| Texas Instruments Incorporated
| USB 3.0 xHCI Host Controller
| Marketing part#   Voltage Range   Package-type   Temperature
| TUSB7340   2.97V - 3.465V   100-Ball RKM QFN   -40 to 105 C
| TUSB7320   2.97V - 3.465V   100-Ball RKM QFN   -40 to 105 C
[IBIS Ver]   4.0
[File name]   tusb7340_20.ibs
[File Rev]   1.0
[Date]   12/02/2010
[Source]   Model built from TISPICE simulations at:
   Texas Instruments Incorporated.
   Analog-eLab, HPA
   12500 TI Blvd
   Dallas, TX -75243
   For Support e-mail: elab_scm_ibis@list.ti.com
[Notes]   Rev 1.0: 12/02/2010
   - Model based on tusb1310.ibs v1.1 09/14/2010 IBIS model.
   - Model generated from simulations in TISPICED
   - For USB2.0, models are included for HS, FS and LS modes
   - For USB3.0, models are included for SATA1, SATA2, No-De-Emphasis
   and De-Emphasis modes
   - USB2 and USB3 Models  matched to TISPICE.
   - C_comp although listed in numerical order of value are obtained from varying
   PVT conditions. For PVT conditions for each specific value refer the buffer
   description under respective [Model]. IBIS model user is responsible for using
   appropriate C_comp to simulate for Signal Integrity
   Where for TUSB7340 & TUSB7320
   Nom PVT:  Nominal process, Typ Temperature, Typ Voltage
   Slow PVT: Weak process, Max Temperature, Min Voltage
   Fast PVT: Strong process, Min Temperatire, Max Voltage
   - ignore warnings related to usb3_WODE, please do not correct this error
   as IBIS parser does not correct IV-VT mismatch with single set of V-T
   waveforms.
   - non-monotonic warnings related to usb2_LS_RC and usb2_LS_R buffers are
   as they are seen in TISPICE simualations
   - [Driver Schedule] is interpreted differently by each system level simulator
   if usual setup with it does not give appropriate results, please
   tie the MAIN and BOOST buffers as per buffer timing description under
   [Driver Schedule] keyword. For example, using HSPICE, refer DE_hspice.sp
   in the correlation report
   - To test USB2/USB3 IBIS models using HSPICE look for spice set up files
   inside the TUSB7340_20 correlation report   \
   - Digital Buffer models are from SR60 standard cell library for TUSB7340
   - Non-Monotonic pulldown warnings related to digital buffers is per
   simulations in TISPICED
[Disclaimer] This product is designed as an aid for customers of Texas Instruments.
   No warranties, either expressed or implied, with respect to this third
   party software (if any) or with respect to its fitness for any
   particular purpose is claimed by Texas Instruments or the author. The
   software (if any) is provided solely on an "as is" basis. The entire
   risk as to its quality and performance is with the customer
[Copyright]   (C)Copyright 2010 Texas Instruments Incorporated.
   All rights reserved.
|   TUSB7340 100-Pin  RKM Package
[Component]   TUSB7340
[Manufacturer]  Texas Instruments Incorporated
[Package]   |100-Pin RKM
|   typ   min   max
R_pkg   0.1421   0.00023   0.2281
L_pkg   1.6573nH   0.0349nH   3.0194nH
C_pkg   0.2292pF   0.0474pF   0.3018pF
[PIN]   signal_name   model_name   R_pin   L_pin   C_pin
A1   VDD11   POWER   0.20633   3.02961nH   0.25239pF
A2   SDA   BI2C33SFZP18   0.19269   2.81314nH   0.26394pF
A3   VDD33   POWER   0.17458   2.52886nH   0.25297pF
A4   VDD11   POWER   0.08243   2.15173nH   0.2545pF
A5   USB_DM_DN4   usb2   0.15088   1.51553nH   0.22318pF
A6   VDD11   POWER   0.14524   2.0709nH   0.20386pF
A7   USB_SSRX_N_DN4   RXP_N   0.14029   1.3887nH   0.19698pF
A8   USB_SSTX_N_DN4   usb3_pcie   0.14108   1.4068nH   0.19507pF
A9   VDD11   POWER   0.07567   1.9807nH   0.23384pF
A10   USB_SSRX_N_DN2   RXP_N   0.15956   1.6073nH   0.22806pF
A11   USB_SSTX_P_DN2   usb3_pcie   0.17543   1.7885nH   0.2505pF
A12   VDD11   POWER   0.09917   2.5372nH   0.33903pF
A13   USB_DM_DN2   usb2   0.21232   2.1735nH   0.28467pF
A14   NC   NC   0.00027   0.0540nH   0.04736pF
A15   GRST#   IC33SHYPBFZP18PU   0.20586   3.0194nH   0.26719pF
A16   VDD11   POWER   0.10263   2.6028nH   0.34437pF
A17   USB_SSTX_P_DN1   usb3_pcie   0.19179   1.8789nH   0.25995pF
A18   USB_SSRX_P_DN1   RXP_N   0.18248   1.8001nH   0.25139pF
A19   VDDA_3P3   POWER   0.17708   2.5649nH   0.24288pF
A20   USB_DP_DN1   usb2   0.17351   1.7226nH   0.23349pF
A21   VDDA_3P3   POWER   0.17352   2.5076nH   0.22324pF
A22   XO   NC   0.17424   2.5197nH   0.23693pF
A23   XI   NC   0.17398   2.5145nH   0.23406pF
A24   R1EXT   NC   0.17821   2.5798nH   0.23553pF
A25   VDDA_3P3   POWER   0.18747   2.7242nH   0.24916pF
A26   NC   NC   0.00027   0.0509nH   0.05748pF
A27   USB_DM_DN3   usb2   0.22809   2.3277nH   0.30184pF
A28   VDD11   POWER   0.10595   2.9231nH   0.33488pF
A29   USB_SSRX_N_DN3   RXP_N   0.18932   1.9225nH   0.26131pF
A30   USB_SSTX_N_DN3   usb3_pcie   0.17333   1.7557nH   0.24429pF
A31   VDD11   POWER   0.15535   2.2185nH   0.20758pF
A32   JTAG_TCK   IC33SHYPBFZP18PD   0.14463   2.0507nH   0.20333pF
A33   VDD11   POWER   0.07029   1.6396nH   0.24364pF
A34   VDD33   POWER   0.07046   1.6451nH   0.24582pF
A35   JTAG_TDI   BC3340DSHYPBFZP18PU  0.14555   2.0652nH   0.20362pF
A36   OVERCUR1#   IC33SHYPBFZP18PU   0.15431   2.2022nH   0.21267pF
A37   OVERCUR2#   IC33SHYPBFZP18PU   0.16904   2.4329nH   0.24474pF
A38   VDD11   POWER   0.19051   2.7701nH   0.24908pF
A39   VDD33   POWER   0.2032   2.9697nH   0.27388pF
A40   PERST#   IC33SHYPBFZP18   0.20159   2.9479nH   0.23728pF
A41   PCIE_TX_N   pcie   0.19448   1.9631nH   0.2971pF
A42   PCIE_RX_N   RXP_N   0.18467   1.8569nH   0.24684pF
A43   NC   NC   0.00027   0.0512nH   0.05626pF
A44   VDDA_3P3   POWER   0.18062   2.6191nH   0.2458pF
A45   PCIE_REFCLK_P   PCIE_REFCLK   0.17476   1.6479nH   0.23691pF
A46   PWRON3#   BC3340DSHYPBFZP18PD  0.17583   2.5449nH   0.23129pF
A47   VDD33   POWER   0.0897   2.1250nH   0.30555pF
A48   PWRON4#   BC3340DSHYPBFZP18PD  0.17959   2.6046nH   0.23816pF
A49   GPIO0   BC3340DSHYPBFZP18PU  0.18549   2.6976nH   0.23704pF
A50   VDD11   POWER   0.09602   2.3280nH   0.32265pF
A51   VDD33   POWER   0.09873   2.4069nH   0.32744pF
A52   AUX_DET   IC33SHYPBFZP18   0.20506   3.0061nH   0.25622pF
B1   VDD11   POWER   0.14492   2.0539nH   0.2197pF
B2   SCL   BI2C33SFZP18   0.13944   1.9647nH   0.26541pF
B3   SM1#   BC3340DSHYPBFZP18   0.13032   1.8225nH   0.25446pF
B4   VDDA_3P3   POWER   0.13458   1.8892nH   0.24905pF
B5   USB_DP_DN4   usb2   0.10866   0.8447nH   0.22343pF
B6   USB_SSRX_P_DN4   RXP_N   0.10465   0.8210nH   0.22203pF
B7   USB_SSTX_P_DN4   usb3_pcie   0.10228   0.7909nH   0.21334pF
B8   NC   NC   0.00023   0.0349nH   0.10524pF
B9   USB_SSRX_P_DN2   RXP_N   0.1157   0.9091nH   0.23967pF
B10   USB_SSTX_N_DN2   usb3_pcie   0.12464   0.9805nH   0.25066pF
B11   VDDA_3P3   POWER   0.13811   1.9442nH   0.26413pF
B12   USB_DP_DN2   usb2   0.15629   1.2845nH   0.24521pF
B13   NC   NC   0.00023   0.0408nH   0.07279pF
B14   FREQSEL   IC33SHYPBFZP18   0.15725   2.2422nH   0.27043pF
B15   USB_SSTX_N_DN1   usb3_pcie   0.1636   1.4218nH   0.29967pF
B16   USB_SSRX_N_DN1   RXP_N   0.14935   1.2666nH   0.27592pF
B17   VDD11   POWER   0.07293   1.6577nH   0.33198pF
B18   USB_DM_DN1   usb2   0.13613   1.1238nH   0.25169pF
B19   VDD11   POWER   0.06764   1.4851nH   0.31674pF
B20   VSS   GND   0.13974   1.9660nH   0.23601pF
B21   VSS_OSC   GND   0.1351   1.8932nH   0.24682pF
B22   VDDA_3P3   POWER   0.13594   1.9051nH   0.24614pF
B23   R1EXTRTN   NC   0.14119   1.9866nH   0.26018pF
B24   VDD11   POWER   0.1513   2.1472nH   0.22651pF
B25   USB_DP_DN3   usb2   0.17263   1.4441nH   0.26411pF
B26   VDDA_3P3   POWER   0.1594   2.2693nH   0.29411pF
B27   USB_SSRX_P_DN3   RXP_N   0.13839   1.1107nH   0.2677pF
B28   USB_SSTX_P_DN3   usb3_pcie   0.12438   0.9769nH   0.25211pF
B29   NC   NC   0.00023   0.0349nH   0.1052pF
B30   JTAG_TMS   IC33SHYPBFZP18PU   0.10418   1.4095nH   0.21511pF
B31   JTAG_TDO   BC3340DSHYPBFZP18PD  0.10232   1.3807nH   0.21783pF
B32   JTAG_RST#   IC33SHYPBFZP18PD   0.10426   1.4108nH   0.21636pF
B33   PWRON1#   BC3340DSHYPBFZP18PD  0.11273   1.5418nH   0.22224pF
B34   PWRON2#   BC3340DSHYPBFZP18PD  0.12373   1.7123nH   0.2463pF
B35   WAKE#   BI2C33SFZP18   0.12963   1.8047nH   0.24689pF
B36   CLKREQ#   BI2C33SFZP18   0.14765   2.0894nH   0.23659pF
B37   VDD11   POWER   0.08651   2.0620nH   0.37191pF
B38   PCIE_TX_P   pcie   0.14718   1.2079nH   0.27639pF
B39   PCIE_RX_P   RXP_N   0.13987   1.1417nH   0.25395pF
B40   VDD11   POWER   0.06941   1.5488nH   0.32287pF
B41   PCIE_REFCLK_N   PCIE_REFCLK   0.14224   1.1238nH   0.25774pF
B42   VDD11   POWER   0.0721   1.6667nH   0.31308pF
B43   OVERCUR3#   IC33SHYPBFZP18PU   0.13888   1.9526nH   0.25276pF
B44   VDD11   POWER   0.07031   1.5227nH   0.32054pF
B45   OVERCUR4#   IC33SHYPBFZP18PU   0.14445   2.0398nH   0.25345pF
B46   GPIO1   BC3340DSHYPBFZP18PU  0.14806   2.0967nH   0.26875pF
B47   GPIO2   BC3340DSHYPBFZP18PU  0.15631   2.2270nH   0.27291pF
B48   GPIO3   BC3340DSHYPBFZP18PU  0.15628   2.2313nH   0.23863pF
[Diff_pin]   inv_pin   vdiff   tdelay_typ   tdelay_min   tdelay_max
B5   A5   880mV  NA NA NA| USB_DP/DM_DN4
B6   A7   1450mV NA NA NA| USB_SSRX_P/N_DN4
B7   A8   2200mV NA NA NA| USB_SSTX_P/N_DN4
B9   A10   1450mV NA NA NA| USB_SSRX_P/N_DN2
A11   B10   2200mV NA NA NA| USB_SSTX_P/N_DN2
B12   A13   880mV  NA NA NA| USB_DP/DM_DN2
A17   B15   2200mV NA NA NA| USB_SSTX_P/N_DN1
A18   B16   1450mV NA NA NA| USB_SSRX_P/N_DN1
A20   B18   880mV  NA NA NA| USB_DP/DM_DN1
B25   A27   880mV  NA NA NA| USB_DP/DM_DN3
B27   A29   1450mV NA NA NA| USB_SSRX_P/N_DN3
B28   A30   2200mV NA NA NA| USB_SSTX_P/N_DN3
B38   A41   2200mV NA NA NA| PCIE_TX_P/N
B39   A42   1450mV NA NA NA| PCIE_RX_P/N
A45   B41   1450mV NA NA NA| PCIE_REFCLK_P/N
[Pin Mapping] pulldown_ref pullup_ref gnd_clamp_ref power_clamp_ref |ext_ref
A1   NC   VDD11BUS|  VDD11
A2   VSSBUS NC   VSSBUS VDD33BUS|  SDA
A3   NC   VDD33BUS|  VDD33
A4   NC   VDD11BUS|  VDD11
A5   VSSBUS VDD33BUS|  USB_DM_DN4
A6   NC   VDD11BUS|  VDD11
A7   VSSBUS VDD11BUS|  USB_SSRX_N_DN4
A8   VSSBUS VDD11BUS|  USB_SSTX_N_DN4
A9   NC   VDD11BUS|  VDD11
A10   VSSBUS VDD11BUS|  USB_SSRX_N_DN2
A11   VSSBUS VDD11BUS|  USB_SSTX_P_DN2
A12   NC   VDD11BUS|  VDD11
A13   VSSBUS VDD33BUS|  USB_DM_DN2
A14   NC   NC   |  NC
A15   NC   NC   VSSBUS VDD33BUS|  GRST#
A16   NC   VDD11BUS|  VDD11
A17   VSSBUS VDD11BUS|  USB_SSTX_P_DN1
A18   VSSBUS VDD11BUS|  USB_SSRX_P_DN1
A19   NC   VDDABUS |  VDDA_3P3
A20   VSSBUS VDD33BUS|  USB_DP_DN1
A21   NC   VDDABUS |  VDDA_3P3
A22   NC   NC   |  XO
A23   NC   NC   |  XI
A24   NC   NC   |  R1EXT
A25   NC   VDDABUS |  VDDA_3P3
A26   NC   NC   |  NC
A27   VSSBUS VDD33BUS|  USB_DM_DN3
A28   NC   VDD11BUS|  VDD11
A29   VSSBUS VDD11BUS|  USB_SSRX_N_DN3
A30   VSSBUS VDD11BUS|  USB_SSTX_N_DN3
A31   NC   VDD11BUS|  VDD11
A32   NC   NC   VSSBUS VDD33BUS|  JTAG_TCK
A33   NC   VDD11BUS|  VDD11
A34   NC   VDD33BUS|  VDD33
A35   VSSBUS VDD33BUS VSSBUS VDD33BUS|  JTAG_TDI
A36   NC   NC   VSSBUS VDD33BUS|  OVERCUR1#
A37   NC   NC   VSSBUS VDD33BUS|  OVERCUR2#
A38   NC   VDD11BUS|  VDD11
A39   NC   VDD33BUS|  VDD33
A40   NC   NC   VSSBUS VDD33BUS|  PERST#
A41   NC   VDD11BUS|  PCIE_TX_N
A42   NC   NC   VSSBUS VDD11BUS|  PCIE_RX_N
A43   NC   NC   |  NC
A44   NC   VDDABUS |  VDDA_3P3
A45   NC   NC   VSSBUS VDD11BUS|  PCIE_REFCLK_P
A46   VSSBUS VDD33BUS VSSBUS VDD33BUS|  PWRON3#
A47   NC   VDD33BUS|  VDD33
A48   VSSBUS VDD33BUS VSSBUS VDD33BUS|  PWRON4#
A49   VSSBUS VDD33BUS VSSBUS VDD33BUS|  GPIO0
A50   NC   VDD11BUS|  VDD11
A51   NC   VDD33BUS|  VDD33
A52   NC   NC   VSSBUS VDD33BUS|  AUX_DET
B1   NC   VDD11BUS|  VDD11
B2   VSSBUS NC   VSSBUS VDD33BUS|  SCL
B3   VSSBUS NC   VSSBUS VDD33BUS|  SM1#
B4   NC   VDDABUS |  VDDA_3P3
B5   VSSBUS VDD33BUS|  USB_DP_DN4
B6   VSSBUS VDD11BUS|  USB_SSRX_P_DN4
B7   VSSBUS VDD11BUS|  USB_SSTX_P_DN4
B8   NC   NC   |  NC
B9   VSSBUS VDD11BUS|  USB_SSRX_P_DN2
B10   VSSBUS VDD11BUS|  USB_SSTX_N_DN2
B11   NC   VDDABUS |  VDDA_3P3
B12   VSSBUS VDD11BUS|  USB_DP_DN2
B13   NC   NC   |  NC
B14   NC   NC   VSSBUS VDD33BUS|  FREQSEL
B15   VSSBUS VDD11BUS|  USB_SSTX_N_DN1
B16   VSSBUS VDD11BUS|  USB_SSRX_N_DN1
B17   NC   VDD11BUS|  VDD11
B18   VSSBUS VDD33BUS|  USB_DM_DN1
B19   NC   VDD11BUS|  VDD11
B20   VSSBUS NC   |  VSS
B21   VSSOSC NC   |  VSS_OSC
B22   NC   VDDABUS |  VDDA_3P3
B23   NC   NC   |  R1EXTRTN
B24   NC   VDD11BUS|  VDD11
B25   VSSBUS VDD11BUS|  USB_DP_DN3
B26   NC   VDDABUS |  VDDA_3P3
B27   VSSBUS VDD11BUS|  USB_SSRX_P_DN3
B28   VSSBUS VDD11BUS|  USB_SSTX_P_DN3
B29   NC   NC   |  NC
B30   NC   NC   VSSBUS VDD33BUS|  JTAG_TMS
B31   VSSBUS VDD33BUS VSSBUS VDD33BUS|  JTAG_TDO
B32   NC   NC   VSSBUS VDD33BUS|  JTAG_RST#
B33   VSSBUS VDD33BUS VSSBUS VDD33BUS|  PWRON1#
B34   VSSBUS VDD33BUS VSSBUS VDD33BUS|  PWRON2#
B35   VSSBUS VDD33BUS VSSBUS VDD33BUS|  WAKE#
B36   VSSBUS VDD33BUS VSSBUS VDD33BUS|  CLKREQ#
B37   NC   VDD11BUS|  VDD11
B38   VSSBUS VDD11BUS|  PCIE_TX_P
B39   VSSBUS VDD11BUS|  PCIE_RX_P
B40   NC   VDD11BUS|  VDD11
B41   NC   NC   VSSBUS VDD11BUS|  PCIE_REFCLK_N
B42   NC   VDD11BUS|  VDD11
B43   NC   NC   VSSBUS VDD33BUS|  OVERCUR3#
B44   NC   VDD11BUS|  VDD11
B45   NC   NC   VSSBUS VDD33BUS|  OVERCUR4#
B46   VSSBUS VDD33BUS VSSBUS VDD33BUS|  GPIO1
B47   VSSBUS VDD33BUS VSSBUS VDD33BUS|  GPIO2
B48   VSSBUS VDD33BUS VSSBUS VDD33BUS|  GPIO3
|   TUSB7320 100-Pin  RKM Package
[Component]   TUSB7320
[Manufacturer]  Texas Instruments Incorporated
[Package]   |100-Pin RKM
|   typ   min   max
R_pkg   0.1421   0.00023   0.2281
L_pkg   1.6573nH   0.0349nH   3.0194nH
C_pkg   0.2292pF   0.0474pF   0.3018pF
[PIN]   signal_name   model_name   R_pin   L_pin   C_pin
A1   VDD11   POWER   0.20633   3.02961nH   0.25239pF
A2   SDA   BI2C33SFZP18   0.19269   2.81314nH   0.26394pF
A3   VDD33   POWER   0.17458   2.52886nH   0.25297pF
A4   VDD11   POWER   0.08243   2.15173nH   0.2545pF
A5   NC   NC   0.15088   1.51553nH   0.22318pF
A6   VDD11   POWER   0.14524   2.0709nH   0.20386pF
A7   NC   NC   0.14029   1.3887nH   0.19698pF
A8   NC   NC   0.14108   1.4068nH   0.19507pF
A9   VDD11   POWER   0.07567   1.9807nH   0.23384pF
A10   USB_SSRX_N_DN2   RXP_N   0.15956   1.6073nH   0.22806pF
A11   USB_SSTX_P_DN2   usb3_pcie   0.17543   1.7885nH   0.2505pF
A12   VDD11   POWER   0.09917   2.5372nH   0.33903pF
A13   USB_DM_DN2   usb2   0.21232   2.1735nH   0.28467pF
A14   NC   NC   0.00027   0.0540nH   0.04736pF
A15   GRST#   IC33SHYPBFZP18PU   0.20586   3.0194nH   0.26719pF
A16   VDD11   POWER   0.10263   2.6028nH   0.34437pF
A17   USB_SSTX_P_DN1   usb3_pcie   0.19179   1.8789nH   0.25995pF
A18   USB_SSRX_P_DN1   RXP_N   0.18248   1.8001nH   0.25139pF
A19   VDDA_3P3   POWER   0.17708   2.5649nH   0.24288pF
A20   USB_DP_DN1   usb2   0.17351   1.7226nH   0.23349pF
A21   VDDA_3P3   POWER   0.17352   2.5076nH   0.22324pF
A22   XO   NC   0.17424   2.5197nH   0.23693pF
A23   XI   NC   0.17398   2.5145nH   0.23406pF
A24   R1EXT   NC   0.17821   2.5798nH   0.23553pF
A25   VDDA_3P3   POWER   0.18747   2.7242nH   0.24916pF
A26   NC   NC   0.00027   0.0509nH   0.05748pF
A27   NC   NC   0.22809   2.3277nH   0.30184pF
A28   VDD11   POWER   0.10595   2.9231nH   0.33488pF
A29   NC   NC   0.18932   1.9225nH   0.26131pF
A30   NC   NC   0.17333   1.7557nH   0.24429pF
A31   VDD11   POWER   0.15535   2.2185nH   0.20758pF
A32   JTAG_TCK   IC33SHYPBFZP18PD   0.14463   2.0507nH   0.20333pF
A33   VDD11   POWER   0.07029   1.6396nH   0.24364pF
A34   VDD33   POWER   0.07046   1.6451nH   0.24582pF
A35   JTAG_TDI   BC3340DSHYPBFZP18PU  0.14555   2.0652nH   0.20362pF
A36   OVERCUR1#   IC33SHYPBFZP18PU   0.15431   2.2022nH   0.21267pF
A37   OVERCUR2#   IC33SHYPBFZP18PU   0.16904   2.4329nH   0.24474pF
A38   VDD11   POWER   0.19051   2.7701nH   0.24908pF
A39   VDD33   POWER   0.2032   2.9697nH   0.27388pF
A40   PERST#   IC33SHYPBFZP18   0.20159   2.9479nH   0.23728pF
A41   PCIE_TX_N   pcie   0.19448   1.9631nH   0.2971pF
A42   PCIE_RX_N   RXP_N   0.18467   1.8569nH   0.24684pF
A43   NC   NC   0.00027   0.0512nH   0.05626pF
A44   VDDA_3P3   POWER   0.18062   2.6191nH   0.2458pF
A45   PCIE_REFCLK_P   PCIE_REFCLK   0.17476   1.6479nH   0.23691pF
A46   NC   NC   0.17583   2.5449nH   0.23129pF
A47   VDD33   POWER   0.0897   2.1250nH   0.30555pF
A48   NC   NC   0.17959   2.6046nH   0.23816pF
A49   GPIO0   BC3340DSHYPBFZP18PU  0.18549   2.6976nH   0.23704pF
A50   VDD11   POWER   0.09602   2.3280nH   0.32265pF
A51   VDD33   POWER   0.09873   2.4069nH   0.32744pF
A52   AUX_DET   IC33SHYPBFZP18   0.20506   3.0061nH   0.25622pF
B1   VDD11   POWER   0.14492   2.0539nH   0.2197pF
B2   SCL   BI2C33SFZP18   0.13944   1.9647nH   0.26541pF
B3   SM1#   BC3340DSHYPBFZP18   0.13032   1.8225nH   0.25446pF
B4   NC   NC   0.13458   1.8892nH   0.24905pF
B5   NC   NC   0.10866   0.8447nH   0.22343pF
B6   NC   NC   0.10465   0.8210nH   0.22203pF
B7   NC   NC   0.10228   0.7909nH   0.21334pF
B8   NC   NC   0.00023   0.0349nH   0.10524pF
B9   USB_SSRX_P_DN2   RXP_N   0.1157   0.9091nH   0.23967pF
B10   USB_SSTX_N_DN2   usb3_pcie   0.12464   0.9805nH   0.25066pF
B11   VDDA_3P3   POWER   0.13811   1.9442nH   0.26413pF
B12   USB_DP_DN2   usb2   0.15629   1.2845nH   0.24521pF
B13   NC   NC   0.00023   0.0408nH   0.07279pF
B14   FREQSEL   IC33SHYPBFZP18   0.15725   2.2422nH   0.27043pF
B15   USB_SSTX_N_DN1   usb3_pcie   0.1636   1.4218nH   0.29967pF
B16   USB_SSRX_N_DN1   RXP_N   0.14935   1.2666nH   0.27592pF
B17   VDD11   POWER   0.07293   1.6577nH   0.33198pF
B18   USB_DM_DN1   usb2   0.13613   1.1238nH   0.25169pF
B19   VDD11   POWER   0.06764   1.4851nH   0.31674pF
B20   VSS   GND   0.13974   1.9660nH   0.23601pF
B21   VSS_OSC   GND   0.1351   1.8932nH   0.24682pF
B22   VDDA_3P3   POWER   0.13594   1.9051nH   0.24614pF
B23   R1EXTRTN   NC   0.14119   1.9866nH   0.26018pF
B24   VDD11   POWER   0.1513   2.1472nH   0.22651pF
B25   NC   NC   0.17263   1.4441nH   0.26411pF
B26   NC   NC   0.1594   2.2693nH   0.29411pF
B27   NC   NC   0.13839   1.1107nH   0.2677pF
B28   NC   NC   0.12438   0.9769nH   0.25211pF
B29   NC   NC   0.00023   0.0349nH   0.1052pF
B30   JTAG_TMS   IC33SHYPBFZP18PU   0.10418   1.4095nH   0.21511pF
B31   JTAG_TDO   BC3340DSHYPBFZP18PD  0.10232   1.3807nH   0.21783pF
B32   JTAG_RST#   IC33SHYPBFZP18PD   0.10426   1.4108nH   0.21636pF
B33   PWRON1#   BC3340DSHYPBFZP18PD  0.11273   1.5418nH   0.22224pF
B34   PWRON2#   BC3340DSHYPBFZP18PD  0.12373   1.7123nH   0.2463pF
B35   WAKE#   BI2C33SFZP18   0.12963   1.8047nH   0.24689pF
B36   CLKREQ#   BI2C33SFZP18   0.14765   2.0894nH   0.23659pF
B37   VDD11   POWER   0.08651   2.0620nH   0.37191pF
B38   PCIE_TX_P   pcie   0.14718   1.2079nH   0.27639pF
B39   PCIE_RX_P   RXP_N   0.13987   1.1417nH   0.25395pF
B40   VDD11   POWER   0.06941   1.5488nH   0.32287pF
B41   PCIE_REFCLK_N   PCIE_REFCLK   0.14224   1.1238nH   0.25774pF
B42   VDD11   POWER   0.0721   1.6667nH   0.31308pF
B43   NC   NC   0.13888   1.9526nH   0.25276pF
B44   VDD11   POWER   0.07031   1.5227nH   0.32054pF
B45   NC   NC   0.14445   2.0398nH   0.25345pF
B46   GPIO1   BC3340DSHYPBFZP18PU  0.14806   2.0967nH   0.26875pF
B47   GPIO2   BC3340DSHYPBFZP18PU  0.15631   2.2270nH   0.27291pF
B48   GPIO3   BC3340DSHYPBFZP18PU  0.15628   2.2313nH   0.23863pF
[Diff_pin]   inv_pin   vdiff   tdelay_typ   tdelay_min   tdelay_max
B9   A10   1450mV NA NA NA| USB_SSRX_P/N_DN2
A11   B10   2200mV NA NA NA| USB_SSTX_P/N_DN2
B12   A13   880mV  NA NA NA| USB_DP/DM_DN2
A17   B15   2200mV NA NA NA| USB_SSTX_P/N_DN1
A18   B16   1450mV NA NA NA| USB_SSRX_P/N_DN1
A20   B18   880mV  NA NA NA| USB_DP/DM_DN1
B38   A41   2200mV NA NA NA| PCIE_TX_P/N
B39   A42   1450mV NA NA NA| PCIE_RX_P/N
A45   B41   1450mV NA NA NA| PCIE_REFCLK_P/N
[Pin Mapping] pulldown_ref pullup_ref gnd_clamp_ref power_clamp_ref |ext_ref
A1   NC   VDD11BUS|  VDD11
A2   VSSBUS NC   VSSBUS VDD33BUS|  SDA
A3   NC   VDD33BUS|  VDD33
A4   NC   VDD11BUS|  VDD11
A5   NC   NC| NC
A6   NC   VDD11BUS|  VDD11
A7   NC   NC| NC
A8   NC   NC| NC
A9   NC   VDD11BUS|  VDD11
A10   VSSBUS VDD11BUS|  USB_SSRX_N_DN2
A11   VSSBUS VDD11BUS|  USB_SSTX_P_DN2
A12   NC   VDD11BUS|  VDD11
A13   VSSBUS VDD33BUS|  USB_DM_DN2
A14   NC   NC   |  NC
A15   NC   NC   VSSBUS VDD33BUS|  GRST#
A16   NC   VDD11BUS|  VDD11
A17   VSSBUS VDD11BUS|  USB_SSTX_P_DN1
A18   VSSBUS VDD11BUS|  USB_SSRX_P_DN1
A19   NC   VDDABUS |  VDDA_3P3
A20   VSSBUS VDD33BUS|  USB_DP_DN1
A21   NC   VDDABUS |  VDDA_3P3
A22   NC   NC   |  XO
A23   NC   NC   |  XI
A24   NC   NC   |  R1EXT
A25   NC   VDDABUS |  VDDA_3P3
A26   NC   NC   |  NC
A27   NC   NC| NC
A28   NC   VDD11BUS|  VDD11
A29   NC   NC| NC
A30   NC   NC| NC
A31   NC   VDD11BUS|  VDD11
A32   NC   NC   VSSBUS VDD33BUS|  JTAG_TCK
A33   NC   VDD11BUS|  VDD11
A34   NC   VDD33BUS|  VDD33
A35   VSSBUS VDD33BUS VSSBUS VDD33BUS|  JTAG_TDI
A36   NC   NC   VSSBUS VDD33BUS|  OVERCUR1#
A37   NC   NC   VSSBUS VDD33BUS|  OVERCUR2#
A38   NC   VDD11BUS|  VDD11
A39   NC   VDD33BUS|  VDD33
A40   NC   NC   VSSBUS VDD33BUS|  PERST#
A41   NC   VDD11BUS|  PCIE_TX_N
A42   NC   NC   VSSBUS VDD11BUS|  PCIE_RX_N
A43   NC   NC   |  NC
A44   NC   VDDABUS |  VDDA_3P3
A45   NC   NC   VSSBUS VDD11BUS|  PCIE_REFCLK_P
A46   NC   NC| NC
A47   NC   VDD33BUS|  VDD33
A48   NC   NC| NC
A49   VSSBUS VDD33BUS VSSBUS VDD33BUS|  GPIO0
A50   NC   VDD11BUS|  VDD11
A51   NC   VDD33BUS|  VDD33
A52   NC   NC   VSSBUS VDD33BUS|  AUX_DET
B1   NC   VDD11BUS|  VDD11
B2   VSSBUS NC   VSSBUS VDD33BUS|  SCL
B3   VSSBUS NC   VSSBUS VDD33BUS|  SM1#
B4   NC   NC| NC
B5   NC   NC| NC
B6   NC   NC| NC
B7   NC   NC| NC
B8   NC   NC   |  NC
B9   VSSBUS VDD11BUS|  USB_SSRX_P_DN2
B10   VSSBUS VDD11BUS|  USB_SSTX_N_DN2
B11   NC   VDDABUS |  VDDA_3P3
B12   VSSBUS VDD11BUS|  USB_DP_DN2
B13   NC   NC   |  NC
B14   NC   NC   VSSBUS VDD33BUS|  FREQSEL
B15   VSSBUS VDD11BUS|  USB_SSTX_N_DN1
B16   VSSBUS VDD11BUS|  USB_SSRX_N_DN1
B17   NC   VDD11BUS|  VDD11
B18   VSSBUS VDD33BUS|  USB_DM_DN1
B19   NC   VDD11BUS|  VDD11
B20   VSSBUS NC   |  VSS
B21   VSSOSC NC   |  VSS_OSC
B22   NC   VDDABUS |  VDDA_3P3
B23   NC   NC   |  R1EXTRTN
B24   NC   VDD11BUS|  VDD11
B25   NC   NC| NC
B26   NC   NC| NC
B27   NC   NC| NC
B28   NC   NC| NC
B29   NC   NC   |  NC
B30   NC   NC   VSSBUS VDD33BUS|  JTAG_TMS
B31   VSSBUS VDD33BUS VSSBUS VDD33BUS|  JTAG_TDO
B32   NC   NC   VSSBUS VDD33BUS|  JTAG_RST#
B33   VSSBUS VDD33BUS VSSBUS VDD33BUS|  PWRON1#
B34   VSSBUS VDD33BUS VSSBUS VDD33BUS|  PWRON2#
B35   VSSBUS VDD33BUS VSSBUS VDD33BUS|  WAKE#
B36   VSSBUS VDD33BUS VSSBUS VDD33BUS|  CLKREQ#
B37   NC   VDD11BUS|  VDD11
B38   VSSBUS VDD11BUS|  PCIE_TX_P
B39   VSSBUS VDD11BUS|  PCIE_RX_P
B40   NC   VDD11BUS|  VDD11
B41   NC   NC   VSSBUS VDD11BUS|  PCIE_REFCLK_N
B42   NC   VDD11BUS|  VDD11
B43   NC   NC| NC
B44   NC   VDD11BUS|  VDD11
B45   NC   NC| NC
B46   VSSBUS VDD33BUS VSSBUS VDD33BUS|  GPIO1
B47   VSSBUS VDD33BUS VSSBUS VDD33BUS|  GPIO2
B48   VSSBUS VDD33BUS VSSBUS VDD33BUS|  GPIO3
[Model Selector] usb2
usb2_HS_R   USB 2.0 High Speed mode, for DP/DM pin 240MHz
usb2_HS_RC   USB 2.0 High Speed mode, for DP/DM pin 240MHz, with Cfixture
usb2_FS_R   USB 2.0 Fast Speed mode, for DP/DM pin 6MHz
usb2_FS_RC   USB 2.0 Fast Speed mode, for DP/DM pin 6MHz, with Cfixture
usb2_LS_RC   USB 2.0 Low  Speed mode, for DP/DM pin 750kHz, with Cfixture
usb2_LS_R   USB 2.0 Low  Speed mode, for DP/DM pin 750kHz
[Model Selector] usb3_pcie
usb3_DE   USB 3.0 De-Emphasis mode, best at 1.25GHz
usb3_WODE   USB 3.0 No De-Emphasis mode, for SSTXP/N 2.5GHz
usb3_SATA1   USB 3.0 SATA1 mode, for SSTXP/N 750MHz
usb3_SATA2   USB 3.0 SATA2 mode, for SSTXP/N 1.5GHz
pcie_GEN2   PCI-E 2.5GHz  GEN2 model
pcie_GEN1   PCI-E 1.25GHz GEN1 model
[Model Selector] pcie
pcie_GEN2   PCI-E 2.5GHz  GEN2 model
pcie_GEN1   PCI-E 1.25GHz GEN1 model
[Model Selector] BC3340DSHYPBFZP18
HYPBFZP18_PI_5P_3P3 BUFFER WITHOUT PULLUP/PULLDOWN & 5% VDDS TOLERANCE
HYPBFZP18_PI_10P_3P3 BUFFER WITHOUT PULLUP/PULLDOWN & 10% VDDS TOLERANCE
[Model Selector] BC3340DSHYPBFZP18PU
FZP18_PU_PI_5P_3P3 BUFFER WITH WEAK PULLUP & 5% VDDS TOLERANCE
FZP18_PU_PI_10P_3P3 BUFFER WITH WEAK PULLUP & 10% VDDS TOLERANCE
[Model Selector] BC3340DSHYPBFZP18PD
FZP18_PD_PI_5P_3P3 BUFFER WITH WEAK PULLDOWN & 5% VDDS TOLERANCE
FZP18_PD_PI_10P_3P3 BUFFER WITH WEAK PULLDOWN & 10% VDDS TOLERANCE
[Model Selector] IC33SHYPBFZP18
C33SHYPBFZP18_10P BUFFER WITHOUT PULLUP/PULLDOWN & 10% VDDS TOLERANCE
C33SHYPBFZP18_5P  BUFFER WITHOUT PULLUP/PULLDOWN & 5% VDDS TOLERANCE
[Model Selector] IC33SHYPBFZP18PD
YPBFZP18_PD_5P BUFFER with WEAK PULLDOWN & 5% VDDS TOLERANCE
YPBFZP18_PD_10P BUFFER with WEAK PULLDOWN & 5% VDDS TOLERANCE
[Model Selector] IC33SHYPBFZP18PU
PBFZP18_PU_5P BUFFER with WEAK PULLUP & 5% VDDS TOLERANCE
PBFZP18_PU_10P BUFFER with WEAK PULLUP & 10% VDDS TOLERANCE
|USB 3.0 De-Emphasis mode, for SSTXP/SSTXN pins 2.5Gbps(1.25GHz to De-Emphasis)
[Model]   usb3_DE
Model_type   Output
Vmeas = 1.1
Vref = 1.1
Rref = 50
|   typ   min   max
|   (TYP PVT)   (Fast PVT) (Slow PVT)
C_comp   0pF   0pF   0pF
[Driver Schedule]
| Model_name   Rise_on_dly Rise_off_dly Fall_on_dly Fall_off_dly
usb3_de_MAIN   0.0nS   0.4ns   0   0.4ns
usb3_de_BOOST   0.0nS   0.2nS   0   0.2nS
[Voltage Range]   1.1   0.99   1.155
[Temperature Range]   27   105   -40
[Pullup Reference]   1.1   0.99   1.155
[Pulldown Reference]   0   0   0
[Power Clamp Reference]   1.1   0.99   1.155
[GND Clamp Reference]   0   0   0
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[Ramp]
R_load = 50
|   typ   min   max
dV/dt_r   0.972315/1.549e-011   0.988218/1.8606e-011   0.957162/1.40763e-011
dV/dt_f   0.972312/7.7916e-012   0.988183/1.21282e-011  0.957081/6.00194e-012
|PCIE GEN2 De-Emphasis mode, for SSTXP/SSTXN pins 5Gbps(2.5GHz to De-Emphasis)
[Model]   pcie_GEN2
Model_type   Output
Vmeas = 1.1
Vref = 1.1
Rref = 50
|   typ   min   max
|   (TYP PVT)   (Fast PVT) (Slow PVT)
C_comp   0pF   0pF   0pF
[Driver Schedule]
| Model_name   Rise_on_dly Rise_off_dly Fall_on_dly Fall_off_dly
usb3_de_MAIN   0.0nS   0.4ns   0   0.4ns
usb3_de_BOOST   0.0nS   0.2nS   0   0.2nS
[Voltage Range]   1.1   0.99   1.155
[Temperature Range]   27   105   -40
[Pullup Reference]   1.1   0.99   1.155
[Pulldown Reference]   0   0   0
[Power Clamp Reference]   1.1   0.99   1.155
[GND Clamp Reference]   0   0   0
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[Ramp]
R_load = 50
|   typ   min   max
dV/dt_r   0.972315/1.549e-011   0.988218/1.8606e-011   0.957162/1.40763e-011
dV/dt_f   0.972312/7.7916e-012   0.988183/1.21282e-011  0.957081/6.00194e-012
|PCIE GEN1 De-Emphasis mode, for SSTXP/SSTXN pins 2.5Gbps(1.25GHz to De-Emphasis)
[Model]   pcie_GEN1
Model_type   Output
Vmeas = 1.1
Vref = 1.1
Rref = 50
|   typ   min   max
|   (TYP PVT)   (Fast PVT) (Slow PVT)
C_comp   0pF   0pF   0pF
[Driver Schedule]
| Model_name   Rise_on_dly Rise_off_dly Fall_on_dly Fall_off_dly
usb3_de_MAIN   0.0nS   0.8ns   0   0.8ns
usb3_de_BOOST   0.0nS   0.4nS   0   0.4nS
[Voltage Range]   1.1   0.99   1.155
[Temperature Range]   27   105   -40
[Pullup Reference]   1.1   0.99   1.155
[Pulldown Reference]   0   0   0
[Power Clamp Reference]   1.1   0.99   1.155
[GND Clamp Reference]   0   0   0
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[Ramp]
R_load = 50
|   typ   min   max
dV/dt_r   0.972315/1.549e-011   0.988218/1.8606e-011   0.957162/1.40763e-011
dV/dt_f   0.972312/7.7916e-012   0.988183/1.21282e-011  0.957081/6.00194e-012
| Models and submodels in the file (29): RXP_N (Input), PCIE_REFCLK (Input), usb2_FS_R (I/O), usb2_FS_RC (I/O), usb2_HS_R (I/O), usb2_HS_RC (I/O), usb2_LS_R (I/O), usb2_LS_RC (I/O), usb3_WODE (Output), usb3_SATA1 (Output), usb3_SATA2 (Output), usb3_DE (Output), usb3_de_MAIN (Output), usb3_de_BOOST (Open_drain), pcie_GEN2 (Output), pcie_GEN1 (Output), HYPBFZP18_PI_5P_3P3 (I/O), HYPBFZP18_PI_10P_3P3 (I/O), FZP18_PU_PI_5P_3P3 (I/O), FZP18_PU_PI_10P_3P3 (I/O), FZP18_PD_PI_5P_3P3 (I/O), FZP18_PD_PI_10P_3P3 (I/O), YPBFZP18_PD_10P (Input), PBFZP18_PU_10P (Input), C33SHYPBFZP18_10P (Input), YPBFZP18_PD_5P (Input), PBFZP18_PU_5P (Input), C33SHYPBFZP18_5P (Input), BI2C33SFZP18 (I/O_open_drain)
